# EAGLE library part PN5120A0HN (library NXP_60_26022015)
Transmission module The PN512 is a highly integrated transceiver IC for contactless communication at 13.56 MHz. This transceiver IC utilizes an outstanding modulation and demodulation concept completely integrated for different kinds of contactless communication methods and protocols at 13.56 MHz. AAL Eindhoven MK
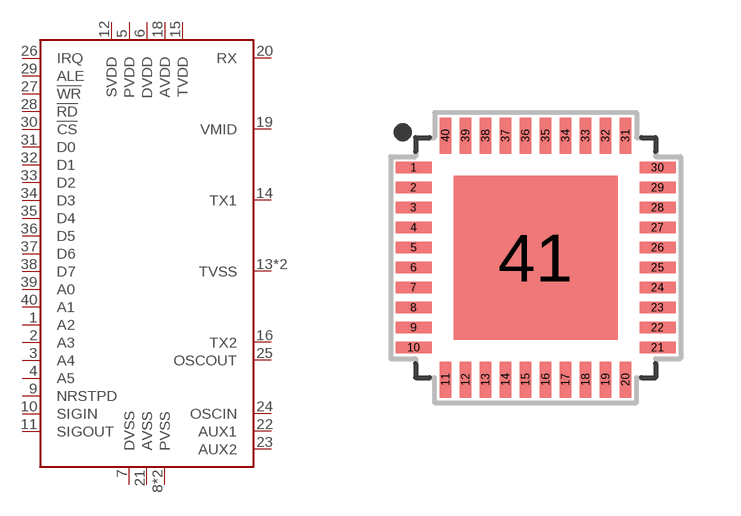
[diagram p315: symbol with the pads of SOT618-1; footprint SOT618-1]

Designator prefix U

## PN5120A0HN  [SOT618-1]
1  A2  in
2  A3  in
3  A4  in
4  A5  in
5  PVDD  pwr
6  DVDD  pwr
7  DVSS  pwr
8  PVSS  pwr
9  NRSTPD  in
10  SIGIN  in
11  SIGOUT  out
12  SVDD  pwr
13  TVSS
14  TX1
15  TVDD  pwr
16  TX2
17  TVSS
18  AVDD  pwr
19  VMID
20  RX
21  AVSS  pwr
22  AUX1  out
23  AUX2  out
24  OSCIN  in
25  OSCOUT  out
26  IRQ  out
27  !WR  in
28  !RD  in
29  ALE  in
30  !CS  in
31  D0
32  D1
33  D2
34  D3
35  D4
36  D5
37  D6
38  D7
39  A0  in
40  A1  in
41  PVSS  pwr

## Footprint SOT618-1 (pad centres in mm)
SOT618-1 HVQFN40: plastic thermal enhanced very thin quad flat package; no leads; 40 terminals; body 6 x 6 x 0.85 mm JEDEC: MO-220 IEC: --
smd 0.9 x 0.29: 1 -3.05,2.25; 2 -3.05,1.75; 3 -3.05,1.25; 4 -3.05,0.75; 5 -3.05,0.25; 6 -3.05,-0.25; 7 -3.05,-0.75; 8 -3.05,-1.25; 9 -3.05,-1.75; 10 -3.05,-2.25; 21 3.05,-2.25; 22 3.05,-1.75; 23 3.05,-1.25; 24 3.05,-0.75; 25 3.05,-0.25; 26 3.05,0.25; 27 3.05,0.75; 28 3.05,1.25; 29 3.05,1.75; 30 3.05,2.25
smd 0.29 x 0.9: 11 -2.25,-3.05; 12 -1.75,-3.05; 13 -1.25,-3.05; 14 -0.75,-3.05; 15 -0.25,-3.05; 16 0.25,-3.05; 17 0.75,-3.05; 18 1.25,-3.05; 19 1.75,-3.05; 20 2.25,-3.05; 31 2.25,3.05; 32 1.75,3.05; 33 1.25,3.05; 34 0.75,3.05; 35 0.25,3.05; 36 -0.25,3.05; 37 -0.75,3.05; 38 -1.25,3.05; 39 -1.75,3.05; 40 -2.25,3.05
smd 4.1 x 4.1: 41 0,0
